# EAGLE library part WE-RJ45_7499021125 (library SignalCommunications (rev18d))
Order Code 7499021125 Design THT xBase-T 10/100 Base-T Ports 1x2 HORIZONTAL Application Standard Tab Position DOWN LED (Left-Right) YELLOW-GREEN EMI Fingers Yes Details see: http://katalog.we-online.de/en/pbs/WE-LAN_RJ45/7499021125? Updated by Yingchun Shan 2016-08-29 2016(C) Würth Elektronik
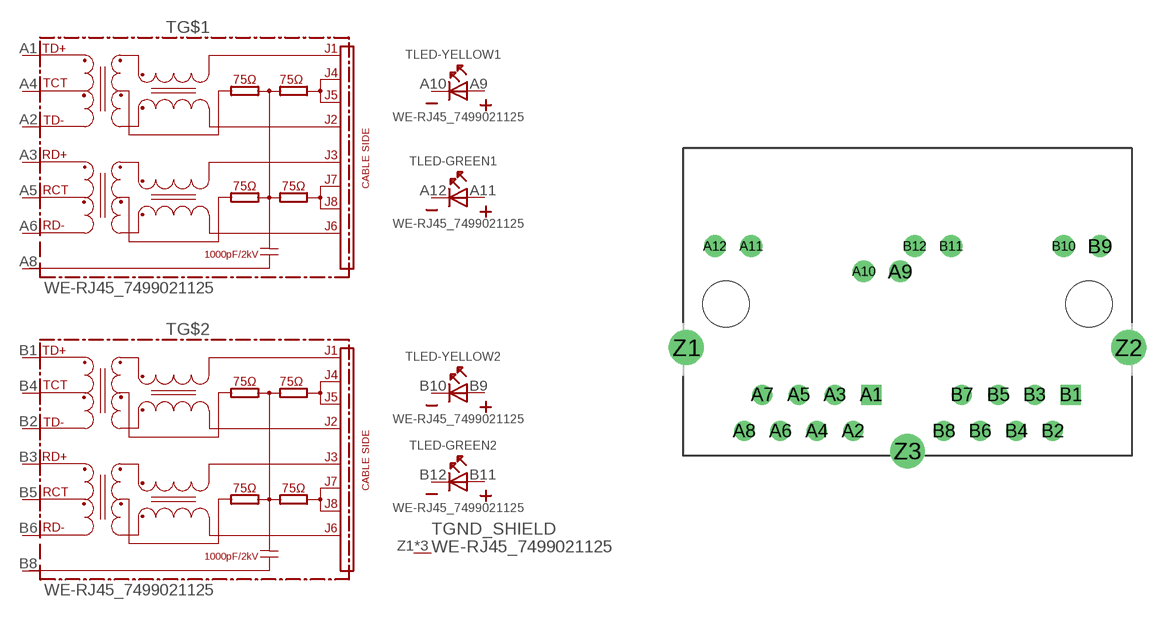
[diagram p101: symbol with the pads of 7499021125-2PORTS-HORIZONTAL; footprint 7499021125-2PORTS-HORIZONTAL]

Designator prefix T; gates LED-YELLOW1=LED2PIN LED-GREEN1=LED2PIN LED-YELLOW2=LED2PIN LED-GREEN2=LED2PIN GND_SHIELD=GND_PIN G$1=74990X-THT-10/100-T G$2=74990X-THT-10/100-T

## WE-RJ45_7499021125 (COMPANY-URL: http://www.we-online.de; CREATED-BY: Christin Zierenner; CREATED-DATE: AUG 2012; DATASHEET-URL: http://katalog.we-online.de/kataloge/eisos/media/pdf/7499021125.pdf; MANUFACTURER: Würth Elektronik eiSos GmbH)  [7499021125-2PORTS-HORIZONTAL]
A1  G$1:TD+
A2  G$1:TD-
A3  G$1:RD+
A4  G$1:TCT
A5  G$1:RCT
A6  G$1:RD-
A8  G$1:8
A9  LED-YELLOW1:A  pas
A10  LED-YELLOW1:K  pas
A11  LED-GREEN1:A  pas
A12  LED-GREEN1:K  pas
B1  G$2:TD+
B2  G$2:TD-
B3  G$2:RD+
B4  G$2:TCT
B5  G$2:RCT
B6  G$2:RD-
B8  G$2:8
B9  LED-YELLOW2:A  pas
B10  LED-YELLOW2:K  pas
B11  LED-GREEN2:A  pas
B12  LED-GREEN2:K  pas
Z1  GND_SHIELD:1  pwr
Z2  GND_SHIELD:1  pwr
Z3  GND_SHIELD:1  pwr

## Footprint 7499021125-2PORTS-HORIZONTAL (pad centres in mm)
MAX HEIGHT=13.50mm PORTS----1X2 HORIZONTAL LED --YES
drill 0.89 square: A1 -2.54,-6.35; B1 11.43,-6.35
drill 0.89: A2 -3.81,-8.89; A3 -5.08,-6.35; A4 -6.35,-8.89; A5 -7.62,-6.35; A6 -8.89,-8.89; A7 -10.16,-6.35; A8 -11.43,-8.89; B2 10.16,-8.89; B3 8.89,-6.35; B4 7.62,-8.89; B5 6.35,-6.35; B6 5.08,-8.89; B7 3.81,-6.35; B8 2.54,-8.89
drill 1.02: A9 -0.51,2.29; A10 -3.05,2.29; A11 -10.93,4.06; A12 -13.47,4.06; B9 13.47,4.06; B10 10.93,4.06; B11 3.05,4.06; B12 0.51,4.06
drill 1.63: Z1 -15.465,-3.05; Z2 15.465,-3.05
drill 1.6: Z3 0,-10.29
hole 3.25 at -12.7,0
hole 3.25 at 12.7,0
